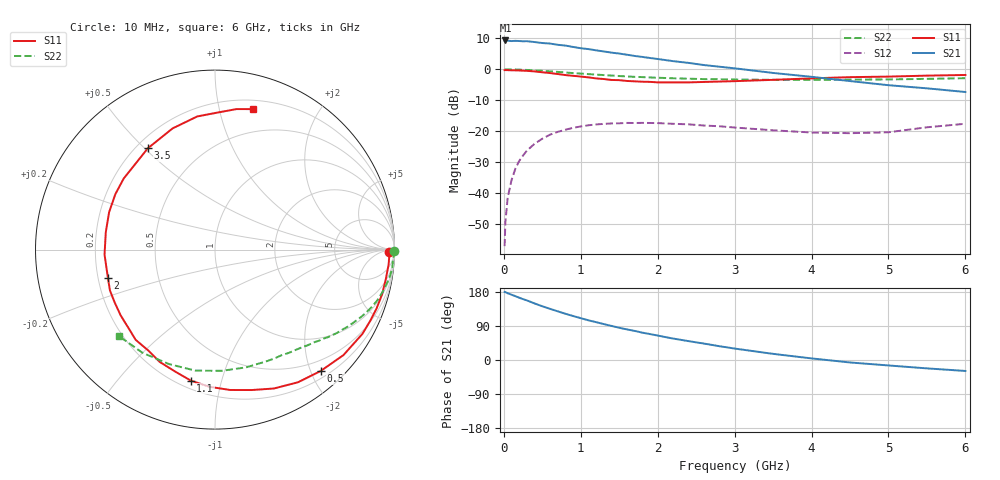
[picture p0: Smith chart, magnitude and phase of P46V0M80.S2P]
! SIEMENS Small Signal Semiconductors
! BFP182
! Si NPN RF Bipolar Junction Transistor in SOT143
! VCE = 6 V  IC = 0.8 mA
! Common Emitter S-Parameters:  March  1996
# GHz  S  MA  R  50
!  f  S11  S21  S12  S22
! GHz  MAG  ANG  MAG  ANG  MAG  ANG  MAG  ANG
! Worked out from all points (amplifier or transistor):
!   36 points, 10 MHz to 6 GHz, reference 50 ohm
!   highest |S21| = 9.3 dB at 20 MHz (marker M1)
!   |S21| within 3 dB of that: start of sweep to 1.153 GHz
!   unconditionally stable (mu >= 1): 2.789 GHz to end of sweep
!   at 250 MHz: K = 0.09, MSG = 18.4 dB, |S12| = -27.8 dB
!   at 1.4 GHz: K = 0.51, MSG = 11.4 dB, |S12| = -17.5 dB
!   at 6 GHz: K = 1.10, MAG = 3.2 dB, |S12| = -17.6 dB
!   S11 on the Smith chart (normalised r, x): 10 MHz: 54, -30; 500 MHz: 0.31, -2.16; 1.1 GHz: 0.25, -0.80; 2 GHz: 0.24, -0.12; 3.5 GHz: 0.25, +0.51; 6 GHz: 0.28, +1.27
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0.01  0.9721 -0.9  2.87 179.6  0.0014 89.2  0.9983 -0.3
0.02  0.9719 -1.8  2.927 179.1  0.0034 83.8  0.997 -0.7
0.05  0.9709 -5.0  2.9 176.2  0.0085 89.9  0.9972 -1.8
0.1  0.9657 -9.8  2.862 172.3  0.0163 81.8  0.9924 -3.5
0.15  0.9638 -15.0  2.884 168.4  0.025 79.8  0.9934 -5.5
0.3  0.9463 -29.7  2.85 157.2  0.0488 71.4  0.9779 -10.7
0.4  0.9261 -39.4  2.758 149.2  0.063 65.3  0.9633 -14.1
0.5  0.8967 -48.9  2.661 141.8  0.076 59.3  0.9479 -17.3
0.6  0.8718 -58.0  2.608 135.0  0.0883 53.9  0.9296 -20.2
0.8  0.8089 -75.3  2.42 122.0  0.1061 43.9  0.8896 -25.6
1.1  0.742 -100.5  2.123 104.7  0.1251 31.3  0.8378 -32.2
1.3  0.6977 -116.1  1.945 94.7  0.1319 24.1  0.808 -36.2
1.5  0.6695 -131.3  1.799 85.1  0.1346 18.0  0.7798 -39.6
1.8  0.6318 -152.3  1.588 72.2  0.1368 10.6  0.7496 -44.4
2  0.6168 -165.4  1.47 64.5  0.1357 6.3  0.7322 -47.6
2.2  0.616 -177.4  1.357 56.6  0.1322 2.6  0.7178 -51.0
2.8  0.6353 150.9  1.104 36.5  0.1207 -5.0  0.6912 -61.3
3.5  0.6771 123.6  0.875 16.2  0.1039 -6.6  0.6786 -75.3
4.5  0.7484 97.6  0.647 -6.5  0.0933 3.2  0.6831 -99.3
5  0.7637 88.9  0.555 -14.4  0.0965 13.4  0.6873 -111.9
5.5  0.792 81.3  0.494 -22.1  0.1161 16.2  0.7028 -125.1
6  0.8114 74.7  0.431 -28.9  0.1324 15.8  0.7193 -137.8
